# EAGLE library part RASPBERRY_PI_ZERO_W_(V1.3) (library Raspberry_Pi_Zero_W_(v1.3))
Raspberry Pi Zero W (v1.3) Single-board Computers Source: Datasheet
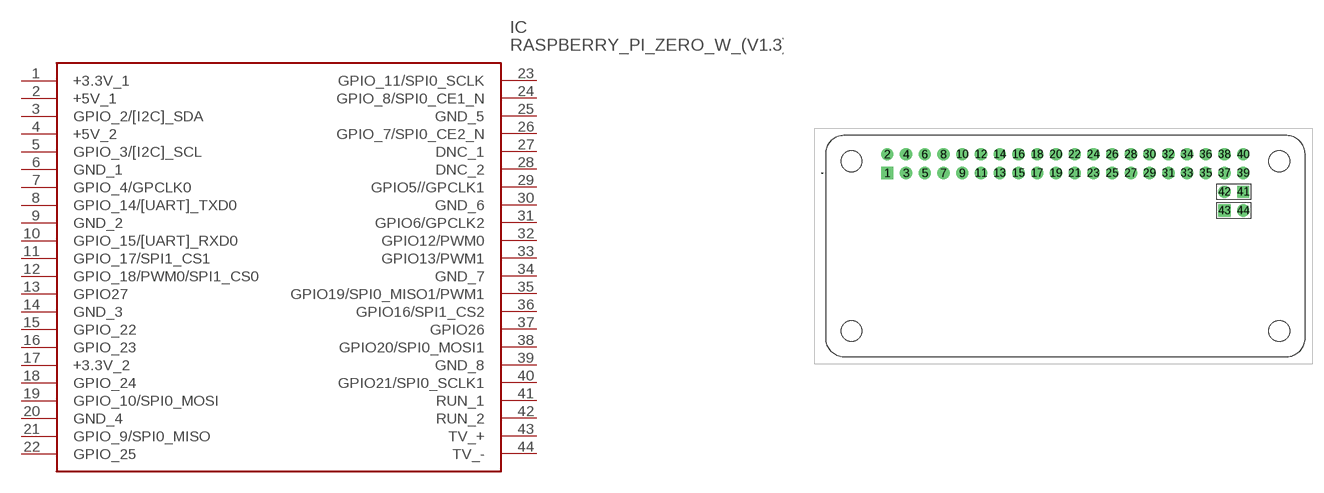
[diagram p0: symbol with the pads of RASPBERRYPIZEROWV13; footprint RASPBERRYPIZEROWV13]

Designator prefix IC

## RASPBERRY_PI_ZERO_W_(V1.3) (Arrow_Part_Number: Raspberry Pi Zero W (v1.3); Description: Raspberry Pi Zero W (v1.3) Single-board Computers; Height: mm; Manufacturer_Name: RASPBERRY-PI; Manufacturer_Part_Number: Raspberry Pi Zero W (v1.3))  [RASPBERRYPIZEROWV13]
1  +3.3V_1
2  +5V_1
3  GPIO_2/[I2C]_SDA
4  +5V_2
5  GPIO_3/[I2C]_SCL
6  GND_1
7  GPIO_4/GPCLK0
8  GPIO_14/[UART]_TXD0
9  GND_2
10  GPIO_15/[UART]_RXD0
11  GPIO_17/SPI1_CS1
12  GPIO_18/PWM0/SPI1_CS0
13  GPIO27
14  GND_3
15  GPIO_22
16  GPIO_23
17  +3.3V_2
18  GPIO_24
19  GPIO_10/SPI0_MOSI
20  GND_4
21  GPIO_9/SPI0_MISO
22  GPIO_25
23  GPIO_11/SPI0_SCLK
24  GPIO_8/SPI0_CE1_N
25  GND_5
26  GPIO_7/SPI0_CE2_N
27  DNC_1
28  DNC_2
29  GPIO5//GPCLK1
30  GND_6
31  GPIO6/GPCLK2
32  GPIO12/PWM0
33  GPIO13/PWM1
34  GND_7
35  GPIO19/SPI0_MISO1/PWM1
36  GPIO16/SPI1_CS2
37  GPIO26
38  GPIO20/SPI0_MOSI1
39  GND_8
40  GPIO21/SPI0_SCLK1
41  RUN_1
42  RUN_2
43  TV_+
44  TV_-

## Footprint RASPBERRYPIZEROWV13 (pad centres in mm)
Raspberry Pi Zero W (v1.3)_1
drill 1.11 pad 1.665 square: 1 -23.885,9.92; 41 24.375,7.38; 43 21.835,4.84
drill 1.11 pad 1.665: 2 -23.885,12.46; 3 -21.345,9.92; 4 -21.345,12.46; 5 -18.805,9.92; 6 -18.805,12.46; 7 -16.265,9.92; 8 -16.265,12.46; 9 -13.725,9.92; 10 -13.725,12.46; 11 -11.185,9.92; 12 -11.185,12.46; 13 -8.645,9.92; 14 -8.645,12.46; 15 -6.105,9.92; 16 -6.105,12.46; 17 -3.565,9.92; 18 -3.565,12.46; 19 -1.025,9.92; 20 -1.025,12.46; 21 1.515,9.92; 22 1.515,12.46; 23 4.055,9.92; 24 4.055,12.46; 25 6.595,9.92; 26 6.595,12.46; 27 9.135,9.92; 28 9.135,12.46; 29 11.675,9.92; 30 11.675,12.46; 31 14.215,9.92; 32 14.215,12.46; 33 16.755,9.92; 34 16.755,12.46; 35 19.295,9.92; 36 19.295,12.46; 37 21.835,9.92; 38 21.835,12.46; 39 24.375,9.92; 40 24.375,12.46; 42 21.835,7.38; 44 24.375,4.84
hole 2.8 at -28.755,11.5
hole 2.8 at -28.755,-11.5
hole 2.8 at 29.245,-11.5
hole 2.8 at 29.245,11.5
